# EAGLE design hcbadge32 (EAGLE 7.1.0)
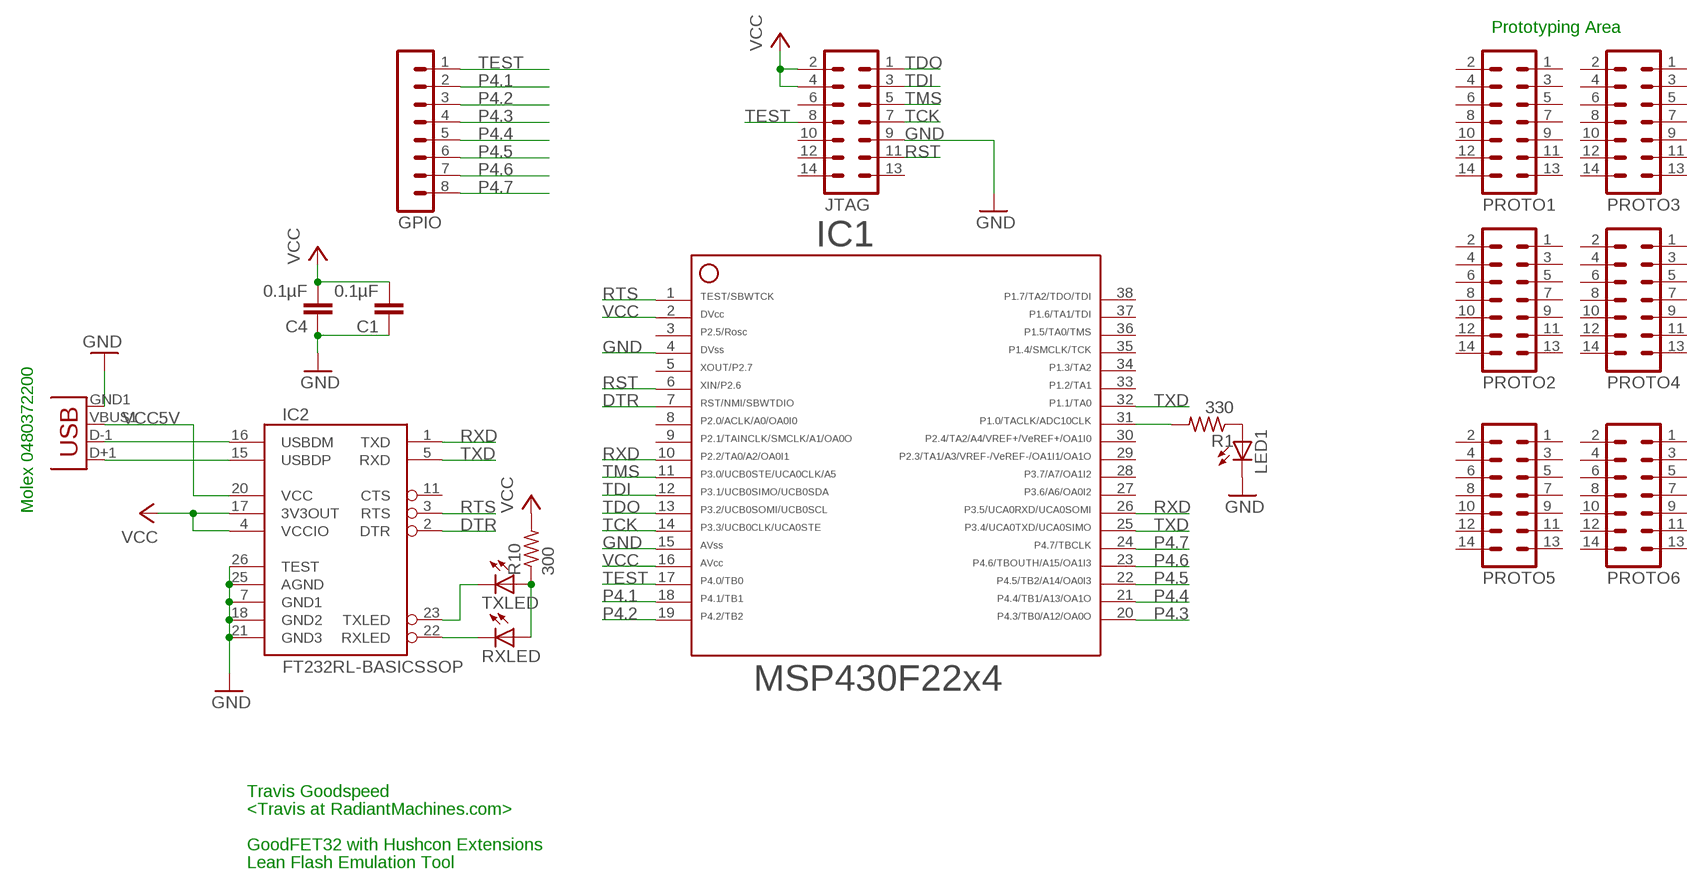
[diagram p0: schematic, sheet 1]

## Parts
C1  0.1µF  C-EUC0603  [C0603]
C4  0.1µF  C-EUC0603  [C0603]
GPIO  MA08-1  [MA08-1]
IC1  F22X4---DA38  [DA38]
IC2  FT232RL-BASICSSOP  [SSOP28DB]
JP1  USBA-SMD-MALE  [USB-A-SMT-MALE]
JTAG  MA07-2  [MA07-2]
LED1  LEDCHIP-LED0603  [CHIP-LED0603]
PROTO1  MA07-2  [MA07-2]
PROTO2  MA07-2  [MA07-2]
PROTO3  MA07-2  [MA07-2]
PROTO4  MA07-2  [MA07-2]
PROTO5  MA07-2  [MA07-2]
PROTO6  MA07-2  [MA07-2]
R1  330  R-US_R0603  [R0603]
R10  300  R-US_R0603  [R0603]
RXLED  LEDCHIP-LED0603  [CHIP-LED0603]
TXLED  LEDCHIP-LED0603  [CHIP-LED0603]

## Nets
DTR: IC1.7 IC2.2(DTR)
GND: C1.1 C4.1 IC1.4 IC1.15 IC2.7(GND1) IC2.18(GND2) IC2.21(GND3) IC2.25(AGND) IC2.26(TEST) JP1.GND1(GND) JTAG.9 LED1.C
N$3: IC2.15(USBDP) JP1.D+1(D+)
N$4: IC2.16(USBDM) JP1.D-1(D-)
N$6: IC2.22(RXLED) RXLED.C
N$7: IC2.23(TXLED) TXLED.C
N$8: R10.1 RXLED.A TXLED.A
N$9: IC1.31 R1.2
N$10: LED1.A R1.1
P4.1: GPIO.2 IC1.18
P4.2: GPIO.3 IC1.19
P4.3: GPIO.4 IC1.20
P4.4: GPIO.5 IC1.21
P4.5: GPIO.6 IC1.22
P4.6: GPIO.7 IC1.23
P4.7: GPIO.8 IC1.24
RST: IC1.6 JTAG.11
RTS: IC1.1 IC2.3(RTS)
RXD: IC1.10 IC1.26 IC2.1(TXD)
TCK: IC1.14 JTAG.7
TDI: IC1.12 JTAG.3
TDO: IC1.13 JTAG.1
TEST: GPIO.1 IC1.17 JTAG.8
TMS: IC1.11 JTAG.5
TXD: IC1.25 IC1.32 IC2.5(RXD)
VCC: C1.2 C4.2 IC1.2 IC1.16 IC2.4(VCCIO) IC2.17(3V3OUT) JTAG.2 JTAG.4 R10.2
VCC5V: IC2.20(VCC) JP1.VBUS1(VBUS)
Unconnected: IC1.3 IC1.5 IC1.8 IC1.9 IC1.27 IC1.28 IC1.29 IC1.30 IC1.33 IC1.34 IC1.35 IC1.36 IC1.37 IC1.38 IC2.11(CTS) JTAG.6 JTAG.10 JTAG.12 JTAG.13 JTAG.14 PROTO1.1 PROTO1.2 PROTO1.3 PROTO1.4 PROTO1.5 PROTO1.6 PROTO1.7 PROTO1.8 PROTO1.9 PROTO1.10 PROTO1.11 PROTO1.12 PROTO1.13 PROTO1.14 PROTO2.1 PROTO2.2 PROTO2.3 PROTO2.4 PROTO2.5 PROTO2.6 PROTO2.7 PROTO2.8 PROTO2.9 PROTO2.10 PROTO2.11 PROTO2.12 PROTO2.13 PROTO2.14 PROTO3.1 PROTO3.2 PROTO3.3 PROTO3.4 PROTO3.5 PROTO3.6 PROTO3.7 PROTO3.8 PROTO3.9 PROTO3.10 PROTO3.11 PROTO3.12 PROTO3.13 PROTO3.14 PROTO4.1 PROTO4.2 PROTO4.3 PROTO4.4 PROTO4.5 PROTO4.6 PROTO4.7 PROTO4.8 PROTO4.9 PROTO4.10 PROTO4.11 PROTO4.12 PROTO4.13 PROTO4.14 PROTO5.1 PROTO5.2 PROTO5.3 PROTO5.4 PROTO5.5 PROTO5.6 PROTO5.7 PROTO5.8 PROTO5.9 PROTO5.10 PROTO5.11 PROTO5.12 PROTO5.13 PROTO5.14 PROTO6.1 PROTO6.2 PROTO6.3 PROTO6.4 PROTO6.5 PROTO6.6 PROTO6.7 PROTO6.8 PROTO6.9 PROTO6.10 PROTO6.11 PROTO6.12 PROTO6.13 PROTO6.14

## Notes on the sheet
- Prototyping Area
- Molex 0480372200
- Travis Goodspeed
- <Travis at RadiantMachines.com>
- GoodFET32 with Hushcon Extensions
- Lean Flash Emulation Tool

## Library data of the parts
C1 C4 = rcl:C-EU: CAPACITOR, European symbol
GPIO = con-lstb:MA08-1: PIN HEADER
IC1 = TI_MSP430_v13:F22X4---DA38: ***MSP430F22x4***DA38
IC2 = SparkFun:FT232RL-BASIC: USB UART This is the simplified version of the FT232RL unit. Only what you need, nothing you don't. Spark Fun Electronics SKU : COM-00650
JP1 = SparkFun-Connectors:USB: USB Connectors USB-B-PTH is fully proven SKU : PRT-00139/CONN-08278 USB-miniB is fully proven SKU : PRT-00587 USB-A-PCB is untested. USB-A-H is throughly reviewed, but untested. Spark Fun Electronics SKU : PRT-00437 USB-B-SMT is throughly reviewed, but untested. Needs silkscreen touching up.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
JTAG PROTO1-PROTO6 = con-lstb:MA07-2: PIN HEADER
LED1 RXLED TXLED = led:LED: LED
R1 R10 = rcl:R-US_: RESISTOR, American symbol

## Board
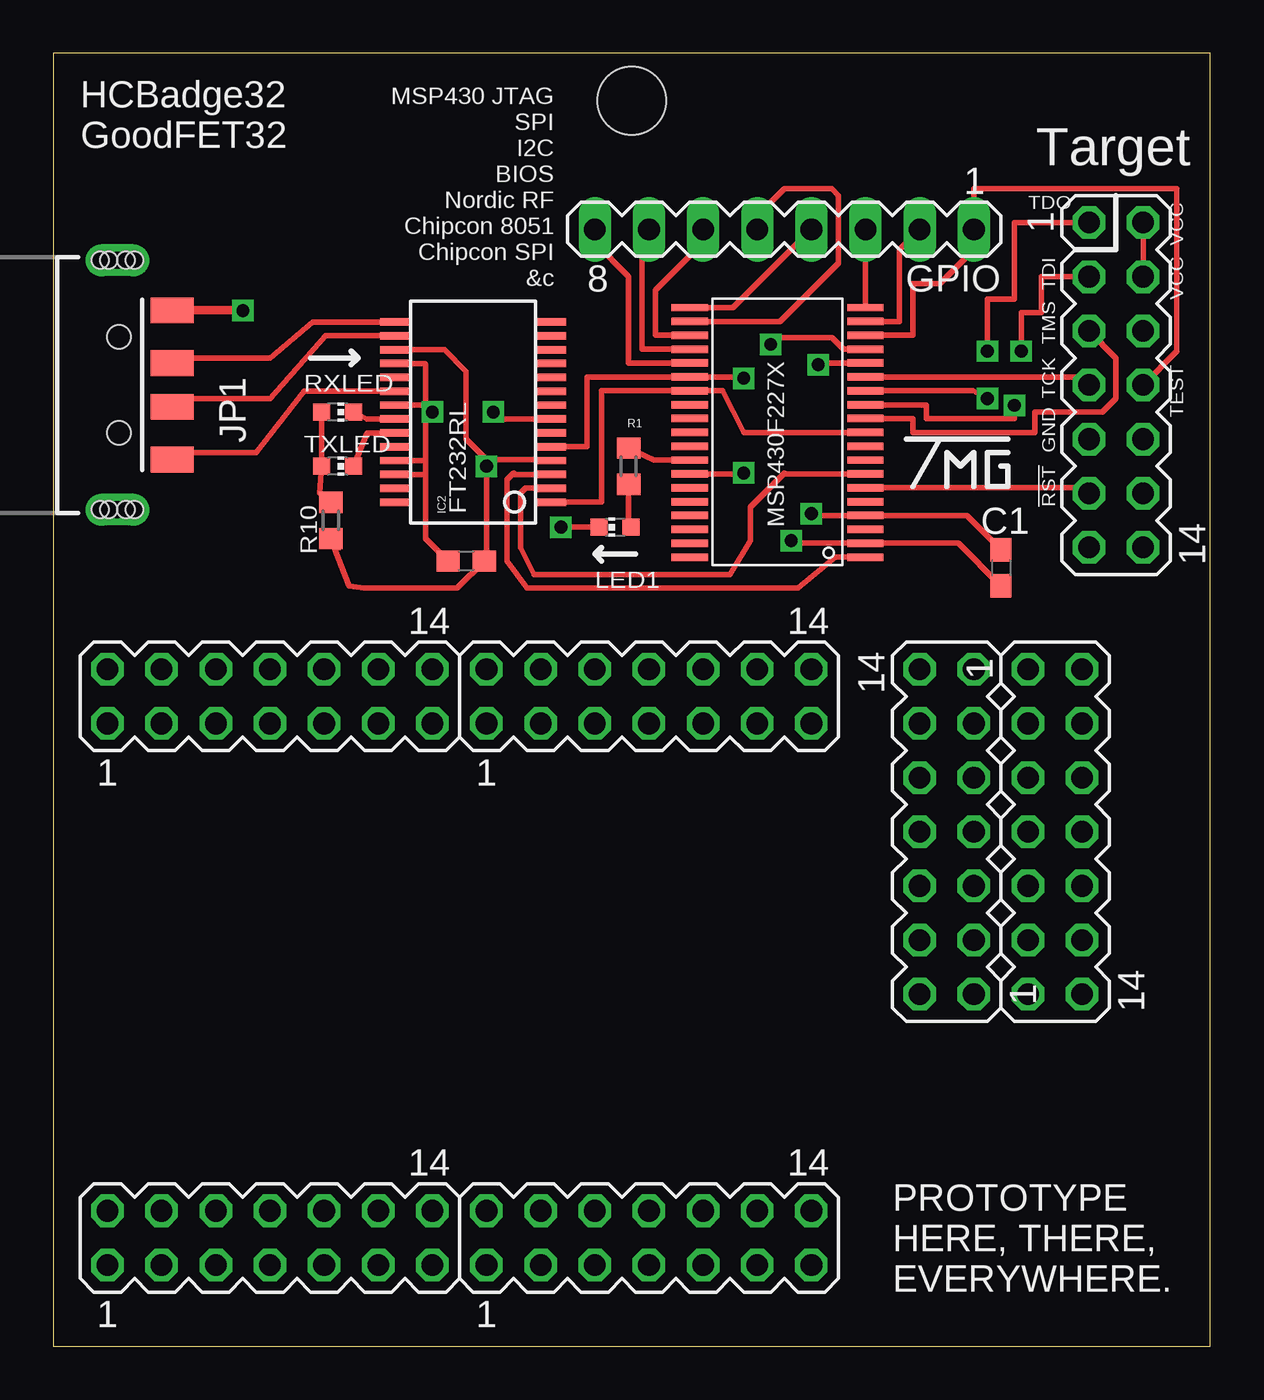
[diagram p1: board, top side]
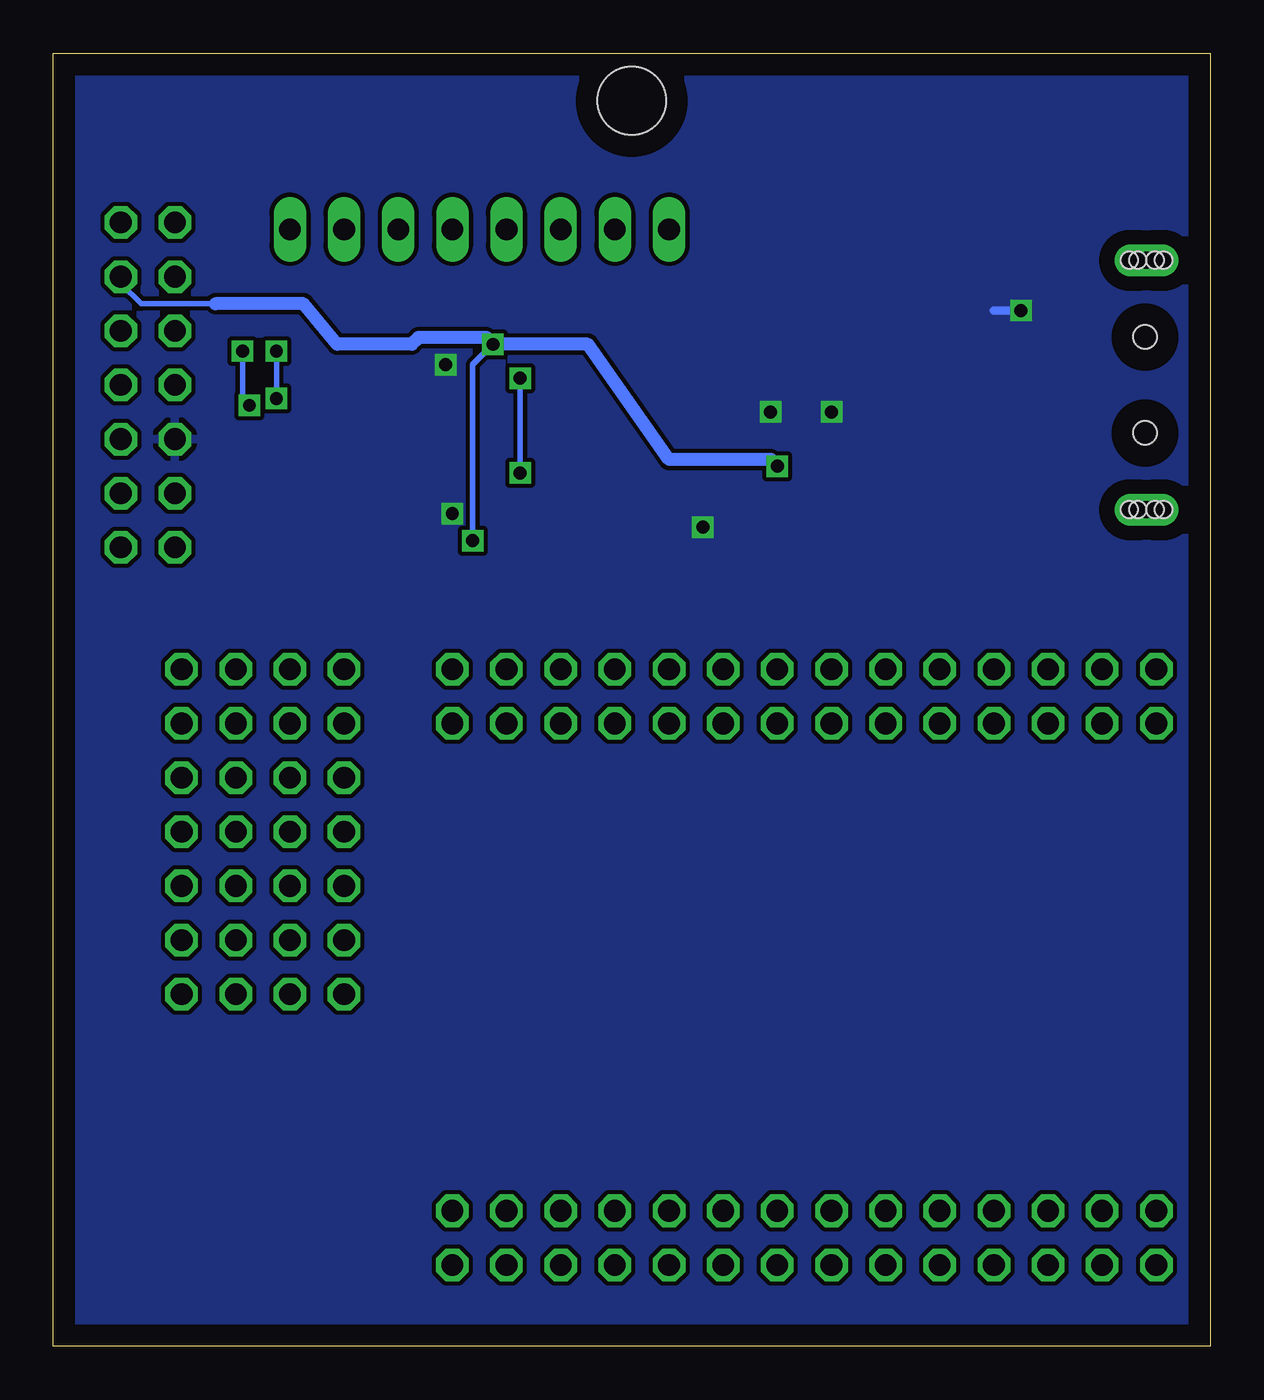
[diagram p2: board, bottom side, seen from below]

Size 54.28 x 60.64 mm. Coordinates in mm from the lower left corner, seen from the top.
Outline: 0,0 54.28,0 54.28,60.64 0,60.64 0,0
Copper layers (1*16): Top 0.035mm / dielectric 1.5mm / Bottom 0.035mm
Design rules "default *": minimum track width 10mil, minimum drill 10mil, track to track 8mil, track to pad 8mil, pad to pad 8mil, via to via 8mil, smd to smd 8mil, copper to edge 40mil, drill to drill 10mil, minimum pad ring 10mil, minimum via ring 8mil, stop-mask expansion 4mil, vias tented up to drill 0mil, thermal gap 10mil
Holes 3.2 mm at 27.14,58.42

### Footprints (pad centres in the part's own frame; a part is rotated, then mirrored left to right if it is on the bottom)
C0603 = smd 1.1 x 1: 1 -0.85,0; 2 0.85,0
MA08-1 = drill 1.016 long: 1 -8.89,0; 2 -6.35,0; 3 -3.81,0; 4 -1.27,0; 5 1.27,0; 6 3.81,0; 7 6.35,0; 8 8.89,0
DA38 = smd 0.35 x 1.705: 1 -5.85,-4.12; 2 -5.2,-4.12; 3 -4.55,-4.12; 4 -3.9,-4.12; 5 -3.25,-4.12; 6 -2.6,-4.12; 7 -1.95,-4.12; 8 -1.3,-4.12; 9 -0.65,-4.12; 10 0,-4.12; 11 0.65,-4.12; 12 1.3,-4.12; 13 1.95,-4.12; 14 2.6,-4.12; 15 3.25,-4.12; 16 3.9,-4.12; 17 4.55,-4.12; 18 5.2,-4.12; 19 5.85,-4.12; 20 5.85,4.12; 21 5.2,4.12; 22 4.55,4.12; 23 3.9,4.12; 24 3.25,4.12; 25 2.6,4.12; 26 1.95,4.12; 27 1.3,4.12; 28 0.65,4.12; 29 0,4.12; 30 -0.65,4.12; 31 -1.3,4.12; 32 -1.95,4.12; 33 -2.6,4.12; 34 -3.25,4.12; 35 -3.9,4.12; 36 -4.55,4.12; 37 -5.2,4.12; 38 -5.85,4.12
SSOP28DB = smd 0.348 x 1.397: 1 -4.225,-3.656; 2 -3.575,-3.656; 3 -2.925,-3.656; 4 -2.275,-3.656; 5 -1.625,-3.656; 6 -0.975,-3.656; 7 -0.325,-3.656; 8 0.325,-3.656; 9 0.975,-3.656; 10 1.625,-3.656; 11 2.275,-3.656; 12 2.925,-3.656; 13 3.575,-3.656; 14 4.225,-3.656; 15 4.225,3.656; 16 3.575,3.656; 17 2.925,3.656; 18 2.275,3.656; 19 1.625,3.656; 20 0.975,3.656; 21 0.325,3.656; 22 -0.325,3.656; 23 -0.975,3.656; 24 -1.625,3.656; 25 -2.275,3.656; 26 -2.925,3.656; 27 -3.575,3.656; 28 -4.225,3.656
USB-A-SMT-MALE = smd 1.2 x 2: D+1 1.027,-3.67; D-1 -1.027,-3.67; GND1 3.5,-3.67; VBUS1 -3.5,-3.67 | drill 0.8 pad 1.5 long: P$1 5.85,-1.1; P$3 -5.85,-1.1 | hole 1.1: 2.25,-1.17; -2.25,-1.17 | hole 0.8: -5.85,-1.5; -5.85,-1.9; -5.85,-0.7; -5.85,-0.3; 5.85,-1.5; 5.85,-1.9; 5.85,-0.7; 5.85,-0.3
MA07-2 = drill 1.016 octagon: 1 -7.62,-1.27; 2 -7.62,1.27; 3 -5.08,-1.27; 4 -5.08,1.27; 5 -2.54,-1.27; 6 -2.54,1.27; 7 0,-1.27; 8 0,1.27; 9 2.54,-1.27; 10 2.54,1.27; 11 5.08,-1.27; 12 5.08,1.27; 13 7.62,-1.27; 14 7.62,1.27
CHIP-LED0603 = smd 0.8 x 0.8: A 0,-0.75; C 0,0.75
R0603 = smd 1 x 1.1: 1 -0.85,0; 2 0.85,0

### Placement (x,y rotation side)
C1  44.45,36.51 270 top
C4  19.37,36.83 0 top
GPIO  34.29,52.39 180 top
IC1  33.97,42.86 90 top
IC2  19.68,43.81 90 top
JP1  1.91,45.09 90 top
JTAG  49.85,45.09 270 top
LED1  26.35,38.42 90 top
PROTO1  10.16,5.08 0 top
PROTO2  27.94,5.08 0 top
PROTO3  10.16,30.48 0 top
PROTO4  27.94,30.48 0 top
PROTO5  41.91,24.13 90 top
PROTO6  46.99,24.13 270 top
R1  26.99,41.27 90 top
R10  13.02,38.73 270 top
RXLED  13.34,43.81 270 top
TXLED  13.34,41.27 270 top

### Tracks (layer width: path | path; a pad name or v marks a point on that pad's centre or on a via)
DTR
  Top 0.254: IC2.2 22.14,40.24 21.91,40.01 21.91,37.47 22.54,36.2 31.75,36.2 32.7,37.78 32.7,39.37 34.29,40.96 34.34,40.91 IC1.7
GND  (via drill 0.6)
  Top 0.254: IC1.15 35.95,46.11 v35.88,46.04 | v35.56,39.05 35.56,38.96 IC1.4 42.85,38.96 C1.1 | IC2.7 20.64,43.49 v20.64,43.81 | IC2.18 17.41,46.09 17.46,46.04 17.46,44.13 | 17.46,40.96 17.46,37.88 C4.1 | 17.46,40.96 17.46,41.59 | 17.46,41.59 17.46,44.13 | IC2.26 17.39,40.89 17.46,40.96 | IC2.25 17.41,41.54 17.46,41.59 | 17.45,44.14 IC2.21 | 17.46,44.13 17.45,44.14 | 17.45,44.14 17.45,43.82 v17.78,43.81 | v23.81,38.42 LED1.C
  Top 0.406: JP1.GND1 v8.89,48.59 v8.89,48.58
  Bottom 0.254: v35.88,46.04 35.56,46.04 | v35.56,39.05 35.24,39.05 | v20.64,43.81 20.32,43.81 | v17.78,43.81 18.1,43.81
  Bottom 0.406: v8.89,48.58 10.16,48.58
  pour Bottom: 0.64,59.69 53.34,59.69 53.66,0.95 0.64,0.95
N$3
  Top 0.254: IC2.15 12.16,48.04 10.16,46.35 5.65,46.35
  Top 0.406: JP1.D+1 5.65,46.11 5.65,46.35
N$4
  Top 0.254: IC2.16 12.78,47.39 10.16,44.45 5.75,44.45
  Top 0.406: JP1.D-1 5.75,44.06 5.75,44.45
N$6
  Top 0.254: IC2.22 14.72,43.49 RXLED.C
N$7
  Top 0.254: IC2.23 14.72,42.84 TXLED.C
N$8
  Top 0.254: RXLED.A TXLED.A 12.48,40.01 R10.1
N$9
  Top 0.254: IC1.31 28.18,41.56 R1.2
N$10
  Top 0.254: R1.1 26.99,38.62 LED1.A
P4.1
  Top 0.254: IC1.18 39.69,48.06 39.69,51.44 GPIO.2
P4.2
  Top 0.254: IC1.19 GPIO.3
P4.3
  Top 0.254: IC1.20 31.89,48.71 GPIO.4
P4.4
  Top 0.254: IC1.21 34.09,48.06 36.83,50.8 36.83,53.98 36.51,54.29 34.29,54.29 33.02,53.02 GPIO.5
P4.5
  Top 0.254: IC1.22 28.26,47.41 28.26,49.53 30.48,51.75 GPIO.6
P4.6
  Top 0.254: IC1.23 27.62,46.76 27.62,51.12 GPIO.7
P4.7
  Top 0.254: IC1.24 26.99,46.11 26.99,50.16 25.4,51.75 GPIO.8
RST
  Top 0.254: IC1.6 48.32,40.26 JTAG.11
RTS
  Top 0.254: IC1.1 36.7,37.01 34.92,35.56 22.23,35.56 21.27,36.83 21.27,40.64 21.59,40.96 21.66,40.89 IC2.3
RXD
  Top 0.254: IC1.10 32.38,42.86 31.39,44.81 IC1.26 25.72,44.81 25.72,39.59 IC2.1
TCK
  Top 0.254: IC1.14 48.2,45.46 JTAG.7
TDI  (via drill 0.6)
  Top 0.254: v45.4,46.67 45.4,48.48 46.35,48.48 46.35,50.16 JTAG.3 | IC1.12 38.09,44.13 40.96,44.13 40.96,43.5 45.09,43.5 v45.09,44.13
  Bottom 0.254: v45.4,46.67 45.4,44.13 v45.09,44.13
TDO  (via drill 0.6)
  Top 0.254: v43.81,46.67 43.81,49.11 45.09,49.11 45.09,52.7 JTAG.1 | v43.81,44.45 43.13,44.81 IC1.13
  Bottom 0.254: v43.81,44.45 v43.81,46.67
TEST
  Top 0.254: IC1.17 40.32,47.41 40.32,49.85 41.59,49.85 43.18,51.44 GPIO.1 43.18,54.29 52.7,54.29 52.7,46.67 JTAG.8
TMS
  Top 0.254: IC1.11 40.32,43.51 40.32,42.86 46.04,42.86 46.04,43.81 49.21,43.81 49.85,44.45 49.85,46.35 JTAG.5
TXD  (via drill 0.6)
  Top 0.254: IC2.5 25.05,42.19 25.05,45.46 IC1.25 32.07,45.46 v32.38,45.4 | IC1.32 32.07,40.91 v32.38,40.96
  Bottom 0.254: v32.38,45.4 v32.38,40.96
VCC  (via drill 0.6)
  Top 0.254: JTAG.4 JTAG.2 | IC2.4 23.29,41.59 20.32,41.59 | IC2.17 18.35,46.74 19.37,45.72 19.37,42.55 20.32,41.59 | 13.44,37.47 R10.2 13.87,35.66 14.61,35.56 18.95,35.56 C4.2 20.32,36.93 v20.32,41.27 20.32,41.59 | IC1.16 37.06,46.76 36.51,47.31 33.97,47.31 v33.66,46.99 | v34.61,37.78 34.73,37.66 IC1.2 42.45,37.66 C1.2
  Bottom 0.254: JTAG.4 51.12,49.85 50.16,48.9 46.67,48.9 | v34.61,37.78 34.61,46.04 v33.66,46.99
  Bottom 0.61: v20.32,41.27 20.64,41.59 25.4,41.59 29.21,46.99 v33.66,46.99 33.97,47.31 37.15,47.31 37.47,46.99 40.96,46.99 42.55,48.9 46.67,48.9
VCC5V
  Top 0.254: IC2.20 11.77,44.79 9.53,41.91 5.4,41.91 5.21,41.91
  Top 0.406: JP1.VBUS1 5.4,41.59 5.4,41.91

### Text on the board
tPlace: HCBadge32 / GoodFET32
tNames: MSP430 JTAG / SPI / I2C / BIOS / Nordic RF / Chipcon 8051 / Chipcon SPI / &c | Target | VCC | TDO | VCC | TDI | TMS | TEST | TCK | GND | FT232RL | !RST | MSP430F227X | PROTOTYPE / HERE, THERE, / EVERYWHERE.

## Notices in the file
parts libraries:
SparkFun-Connectors: Licensing: CC v3.0 Share-Alike You are welcome to use this library for commercial purposes.
